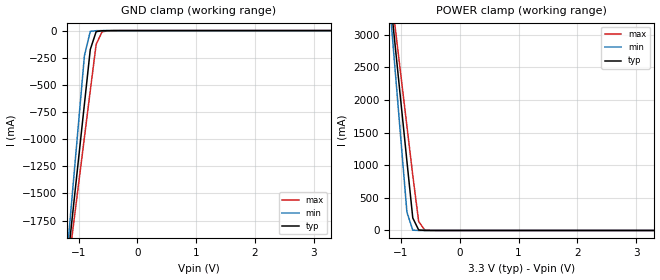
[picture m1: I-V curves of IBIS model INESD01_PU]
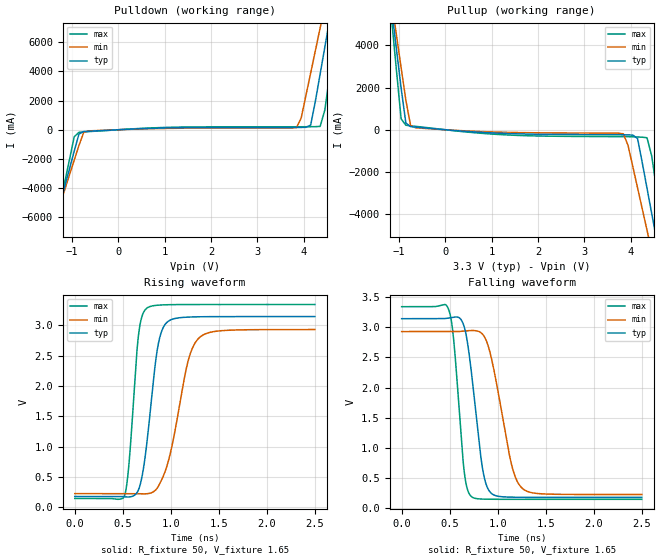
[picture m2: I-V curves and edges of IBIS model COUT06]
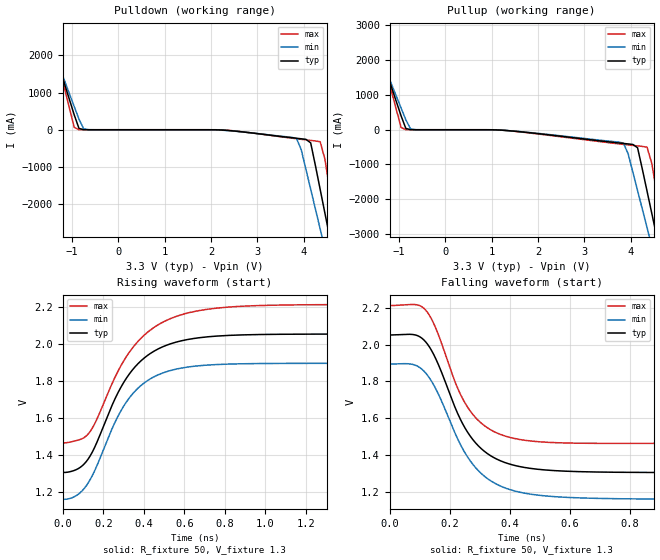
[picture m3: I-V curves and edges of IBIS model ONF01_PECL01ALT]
|   This file is an IBIS representation of the   |
|   Integrated Devices Technology, Inc.   |
|   ICS84329B-01   |
|700MHZ, LOW JITTER,CRYSTAL-TO-3.3V DIFFERENTIAL LVPECL FREQUENCY SYNTHESIZER|
[IBIS Ver]   4.1
[File name]   84329b_01_3v3.ibs
[File Rev]   1.0
[Date]   5 Jan 2009 | Last modified
|   Apr 20 2005 | Generated
[Source]   Originated at Integrated Devices Technology, Inc.
[Disclaimer]
IDT hereby grants the user of this IBIS model a non-exclusive,
nontransferable license to use this IBIS model under the following terms.
Before using this IBIS model, the user should read this license.
If the user does not accept these terms,  the IBIS model should be
returned to IDT within 30 days.
   The user is granted this license only to use the IBIS model and
is not granted rights to sell, load, rent, lease or license the IBIS
model in whole or in part, or in modified form to anyone other than
user. User may modify the IBIS model to suit its specific
applications but rights to derivative works and such modifications
shall belong to IDT.
   This IBIS model is provided on an "AS IS" basis and IDT makes
absolutely no warranty with respect to the information contained
herein. IDT DISCLAIMS AND CUSTOMER WAIVES ALL WARRANTIES, EXPRESS
OR IMPLIED, INCLUDING WARRANTIES OF MERCHANTABILITY OR FITNESS FOR
A PARTICULAR PURPOSE. The entire risk as to quality and performance
is with the Customer. ACCORDINGLY, IN NO EVENT SHALL THE COMPANY BE
LIABLE FOR ANY DAMAGES, WHETHER IN CONTRACT OR TORT,INCLUDING ANY
LOST PROFITS OR OTHER INCIDENTAL, CONSEQUENTIAL, EXEMPLARY, OR
PUNITIVE DAMAGES ARISING OUT OF THE USE OR APPLICATION OF THE IBIS
model provided in this package. Further, IDT reserves the right to
make changes without notice to any product herein to improve
reliability, function, or design. IDT does not convey any license
under patent rights or any other intellectual property rights,
including those of third parties.
   IDT is not obligated to provide maintenance or support
for the licensed IBIS model.
[Copyright]   Copyright 2005 by Integrated Devices Technology, Inc.
[Component]   ICS84329BM-01
[Manufacturer] Integrated Devices Technology, Inc.
[Package]
|SOIC 28 Lead
|   typ   min   max
R_pkg   57.15m   45.4m   68.9m
L_pkg   4.051nH   2.187nH   5.914nH
C_pkg   0.796pF   0.419pF   1.173pF
[Pin] signal_name  model_name   R_pin   L_pin   C_pin
1   M0   INESD01_PU   68.9m   5.914n   1.173p
2   M1   INESD01_PU   65.0m   5.288n   1.044p
3   M2   INESD01_PU   61.1m   4.668n   0.919p
4   M3   INESD01_PU   57.2m   4.048n   0.794p
5   M4   INESD01_PU   53.2m   3.428n   0.669p
6   M5   INESD01_PU   49.3m   2.808n   0.544p
7   M6   INESD01_PU   45.4m   2.187n   0.419p
8   M7   INESD01_PU   45.4m   2.187n   0.419p
9   M8   INESD01_PU   49.3m   2.808n   0.544p
10   N0   INESD01_PU   53.2m   3.428n   0.669p
11   N1   INESD01_PU   57.2m   4.048n   0.794p
12   VEE   GND   61.1m   4.668n   0.919p
13   TEST   COUT06   65.0m   5.288n   1.044p
14   VCC   POWER   68.9m   5.914n   1.173p
15   VEE   GND   68.9m   5.914n   1.173p
16   nFOUT   ONF01_PECL01ALT   65.0m   5.288n   1.044p
17   FOUT   ONF01_PECL01ALT   61.1m   4.668n   0.919p
18   VCC   POWER   57.2m   4.048n   0.794p
19   S_CLOCK   INESD01_PD   53.2m   3.428n   0.669p
20   S_DATA   INESD01_PD   49.3m   2.808n   0.544p
21   S_LOAD   INESD01_PD   45.4m   2.187n   0.419p
22   VCCA   POWER   45.4m   2.187n   0.419p
23   NC   NC   49.3m   2.808n   0.544p
24   NC   NC   53.2m   3.428n   0.669p
25   XTAL_IN   NC   57.2m   4.048n   0.794p
26   XTAL_OUT   NC   61.1m   4.668n   0.919p
27   VCC   POWER   65.0m   5.288n   1.044p
28   nP_LOAD   INESD01_PU   68.9m   5.914n   1.173p
[Diff Pin]  inv_pin  vdiff tdelay_typ tdelay_min  tdelay_max
17   16   NA   0  0  0
[Component]   ICS84329BV-01
[Manufacturer] Integrated Devices Technology, Inc.
[Package]
|PLCC 28 Pin
|   typ   min   max
R_pkg   53.15m   49.2m   57.1m
L_pkg   3.123nH   2.878nH   3.368nH
C_pkg   0.65pF   0.632pF   0.667pF
[Pin] signal_name   model_name   R_pin   L_pin   C_pin
1   VCCA   POWER   49.2m   2.878n   0.632p
2   NC   NC   51.2m   3.038n   0.643p
3   NC   NC   53.8m   3.201n   0.655p
4   XTAL_IN   NC   57.1m   3.368n   0.667p
5   XTAL_OUT   NC   57.1m   3.368n   0.667p
6   VCC   POWER   53.8m   3.201n   0.655p
7   nP_LOAD   INESD01_PU   51.2m   3.038n   0.643p
8   M0   INESD01_PU   49.2m   2.878n   0.632p
9   M1   INESD01_PU   51.2m   3.038n   0.643p
10   M2   INESD01_PU   53.8m   3.201n   0.655p
11   M3   INESD01_PU   57.1m   3.368n   0.667p
12   M4   INESD01_PU   57.1m   3.368n   0.667p
13   M5   INESD01_PU   53.8m   3.201n   0.655p
14   M6   INESD01_PU   51.2m   3.038n   0.643p
15   M7   INESD01_PU   49.2m   2.878n   0.632p
16   M8   INESD01_PU   51.2m   3.038n   0.643p
17   N0   INESD01_PU   53.8m   3.201n   0.655p
18   N1   INESD01_PU   57.1m   3.368n   0.667p
19   VEE   GND   57.1m   3.368n   0.667p
20   TEST   COUT06   53.8m   3.201n   0.655p
21   VCC   POWER   51.2m   3.038n   0.643p
22   VEE   GND   49.2m   2.878n   0.632p
23   nFOUT   ONF01_PECL01ALT   51.2m   3.038n   0.643p
24   FOUT   ONF01_PECL01ALT   53.8m   3.201n   0.655p
25   VCC   POWER   57.1m   3.368n   0.667p
26   S_CLOCK   INESD01_PD   57.1m   3.368n   0.667p
27   S_DATA   INESD01_PD   53.8m   3.201n   0.655p
28   S_LOAD   INESD01_PD   51.2m   3.038n   0.643p
[Diff Pin]  inv_pin  vdiff tdelay_typ tdelay_min  tdelay_max
24   23   NA   0  0  0
| Models and submodels in the file (4): INESD01_PU (Input), COUT06 (Output), ONF01_PECL01ALT (Output_ECL), INESD01_PD (Input)
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[Model]   INESD01_PU
Model_type   Input
Polarity   Non-Inverting
Vinl = 0.8V
Vinh = 2.0V
|   typ   min   max
C_comp   2pF   1.5pF   2.5pF
|   typ   min   max
[Voltage range]  3.3V   3.15V   3.45V
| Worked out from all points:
|   GND clamp passes 1 mA (typ) near -0.55 V on its own axis
|   POWER clamp passes 1 mA (typ) near -0.61 V on its own axis
[GND_clamp]
|Voltage   I(typ)   I(min)   I(max)
-3.3V     -12.83A    -15.14A    -11.37A
-1.2V     -2.195A    -2.092A    -2.281A
-1.1V     -1.689A    -1.472A    -1.849A
-900mV    -678.5mA   -232.7mA   -984.8mA
-800mV    -174mA     -7.237mA   -553.3mA
-700mV    -9.767mA   -1.114mA   -126.1mA
-600mV    -1.7mA     -240.1uA   -11.15mA
-300mV    -81.66uA   -67.79uA   -163.4uA
3.3V      1.866nA    1.113pA    239.1nA
[POWER_clamp]
|Voltage   I(typ)   I(min)   I(max)
-3.3V     22.38A     26.45A     19.82A
-1.2V     3.723A     3.545A     3.874A
-1.1V     2.836A     2.457A     3.116A
-1V       1.949A     1.369A     2.358A
-900mV    1.063A     281mA      1.601A
-800mV    191.5mA    5.012mA    843.9mA
-700mV    8.032mA    142.2uA    138.3mA
-600mV    607uA      17.63uA    10.62mA
-400mV    16.32uA    7.545uA    335.9uA
3.3V      -71.13uA   -62.11uA   -78.26uA
[Model]   COUT06
Model_type   Output
Polarity   Non-Inverting
|   typ   min   max
C_comp   2pF   1.5pF   2.5pF
Vmeas = 1.65V
Rref = 50
Vref = 1.65V
|   typ   min   max
[Voltage range]   3.3V   3.135V   3.465V
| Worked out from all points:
|   slope of the pulldown table from 0 to 0.495 V, typ, clamps not added: 6.88 ohm
|   slope of the pullup table from 0 to 0.495 V, typ, clamps not added: 5.83 ohm
|   rising waveform, R_fixture 50, V_fixture 1.65: 20-80 % time 127ps typ, 201ps min, 86.3ps max; typ from 0.181 V to 3.14 V
|   falling waveform, R_fixture 50, V_fixture 1.65: 20-80 % time 128ps typ, 189ps min, 92.7ps max; typ from 3.14 V to 0.181 V
[pulldown]
|Voltage   I (typ)   I (min)   I (max)
-3.3V     -29.26A    -25.24A    -35.98A
-1.463V   -7.508A    -7.113A    -8.217A
-1.361V   -6.298A    -6.106A    -6.67A
-952.6mV  -1.454A    -2.076A    -481.7mA
-850.5mV  -293.8mA   -1.069A    -175.5mA
-646.4mV  -102mA     -81.18mA   -129.6mA
3.844V    159mA      144.7mA    203.8mA
4.151V    319.9mA    3.884A     206.6mA
4.355V    3.815A     6.961A     228.9mA
4.559V    7.514A     10.04A     3.725A
4.763V    11.22A     13.12A     8.46A
6.6V      44.81A     41.05A     51.4A
[pullup]
|Voltage   I (typ)   I (min)   I (max)
-3.3V     44.73A     38.54A     55.09A
-1.157V   5.7A       6.046A     5.224A
-1.055V   3.84A      4.498A     2.846A
-952.6mV  1.979A     2.95A      516.9mA
-850.5mV  318.6mA    1.402A     214.1mA
-748.5mV  147.6mA    205.9mA    188.2mA
3.844V    -239.7mA   -193.2mA   -328.3mA
4.151V    -416.1mA   -2.755A    -342.5mA
4.355V    -2.772A    -4.758A    -379.9mA
4.559V    -5.183A    -6.764A    -2.792A
4.763V    -7.594A    -8.771A    -5.873A
6.6V      -29.3A     -26.85A    -33.6A
[Ramp]
|   typ   min   max
dV/dt_r   2.374/0.197n   2.162/0.318n   2.564/0.133n
dV/dt_f   2.390/0.193n   2.173/0.283n   2.581/0.140n
[Rising Waveform]
R_fixture = 50
V_fixture = 1.65
V_fixture_max = 1.7325
V_fixture_min = 1.56
C_fixture = 0.0p
| Time   typ   min   max
0s        180.7mV    228.1mV    148.5mV
517.1ps   175.7mV    228.2mV    190.5mV
564.8ps   172.8mV    228.4mV    725.4mV
662.6ps   287.2mV    227.2mV    2.825V
748ps     1.026V     225.5mV    3.276V
863.4ps   2.637V     331.6mV    3.328V
971.4ps   3.061V     746.1mV    3.336V
1.175ns   3.132V     2.376V     3.339V
1.298ns   3.137V     2.795V     3.339V
2.5ns     3.141V     2.927V     3.339V
[Falling Waveform]
R_fixture = 50
V_fixture = 1.65
V_fixture_max = 1.7325
V_fixture_min = 1.56
C_fixture = 0.0p
| Time   typ   min   max
0s        3.141V     2.927V     3.339V
489.5ps   3.152V     2.927V     3.292V
542.2ps   3.165V     2.927V     2.783V
652.6ps   2.999V     2.936V     592.4mV
727.9ps   2.231V     2.945V     192.6mV
828.3ps   806.2mV    2.905V     153.4mV
888.5ps   358.5mV    2.748V     150.6mV
1.142ns   184.2mV    738.8mV    148.6mV
1.252ns   181.9mV    336.5mV    148.5mV
2.5ns     180.7mV    228.1mV    148.5mV
[Model]   ONF01_PECL01ALT
Model_type  Output_ECL
Polarity   Non-Inverting
Vmeas = 1.636
Rref = 50
Cref = 0
Vref = 1.3
|Variable  typ   min   max
C_comp   2p   1.5p   2.5p
[Voltage Range]   3.3   3.135   3.465
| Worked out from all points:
|   rising waveform, R_fixture 50, V_fixture 1.3: 20-80 % time 218ps typ, 206ps min, 242ps max; typ from 1.31 V to 2.05 V
|   falling waveform, R_fixture 50, V_fixture 1.3: 20-80 % time 134ps typ, 143ps min, 120ps max; typ from 2.05 V to 1.31 V
| Open source, no load
|  Voltage   I(typ)   I(min)   I(max)
[Pullup]
-3.3V     9.786A     8.45A      12.03A
-1.667V   3.247A     2.997A     3.691A
-1.565V   2.839A     2.657A     3.17A
-952.6mV  398mA      622.1mA    64.71mA
-850.5mV  36.63mA    284.2mA    1.532mA
-646.4mV  229.3uA    1.611mA    19.07uA
3.844V    -394.4mA   -383.6mA   -421.3mA
4.151V    -517.8mA   -1.749A    -465.4mA
4.355V    -1.764A    -2.812A    -500.3mA
4.559V    -3.036A    -3.875A    -1.773A
4.763V    -4.308A    -4.937A    -3.393A
6.6V      -15.79A    -14.52A    -18.03A
[Pulldown]
-3.3V     9.786A     8.45A      12.03A
-1.565V   2.839A     2.657A     3.17A
-1.463V   2.432A     2.317A     2.65A
-952.6mV  398mA      622.1mA    64.71mA
-850.5mV  36.63mA    284.2mA    1.532mA
-646.4mV  229.3uA    1.611mA    19.07uA
3.844V    -229.1mA   -232.1mA   -241.8mA
4.151V    -352.7mA   -1.598A    -286.7mA
4.355V    -1.599A    -2.66A     -322.1mA
4.559V    -2.871A    -3.722A    -1.595A
4.763V    -4.144A    -4.785A    -3.217A
6.6V      -15.69A    -14.41A    -17.97A
[Ramp]
|   typ   min   max
dV/dt_r   0.45V/0.37ns   0.45V/0.405ns   0.45V/0.27ns
dV/dt_f   0.45V/0.37ns   0.45V/0.405ns   0.45V/0.27ns
R_load =   50.0000
[Rising Waveform]
R_fixture = 50
V_fixture = 1.3   | VCC_typ - 2V
V_fixture_max = 1.465   | VCC_max - 2V
V_fixture_min = 1.135   | VCC_min - 2V
C_fixture = 0.0p
| Time   typ   min   max
0s        1.306V     1.161V     1.465V
70ps      1.323V     1.183V     1.479V
128ps     1.383V     1.254V     1.517V
258ps     1.703V     1.577V     1.819V
316ps     1.817V     1.689V     1.934V
398ps     1.919V     1.785V     2.042V
504ps     1.988V     1.846V     2.121V
658ps     2.03V      1.879V     2.175V
875ps     2.047V     1.891V     2.201V
2ns       2.052V     1.894V     2.211V
[Falling Waveform]
R_fixture = 50
V_fixture = 1.3   | VCC_typ - 2V
V_fixture_max = 1.465   | VCC_max - 2V
V_fixture_min = 1.135   | VCC_min - 2V
C_fixture = 0.0p
0s        2.052V     1.894V     2.211V
76ps      2.055V     1.893V     2.217V
118ps     2.018V     1.85V      2.19V
150ps     1.936V     1.772V     2.103V
222ps     1.644V     1.505V     1.782V
264ps     1.514V     1.38V      1.65V
326ps     1.409V     1.274V     1.549V
410ps     1.348V     1.21V      1.493V
708ps     1.309V     1.166V     1.465V
2ns       1.306V     1.161V     1.465V
